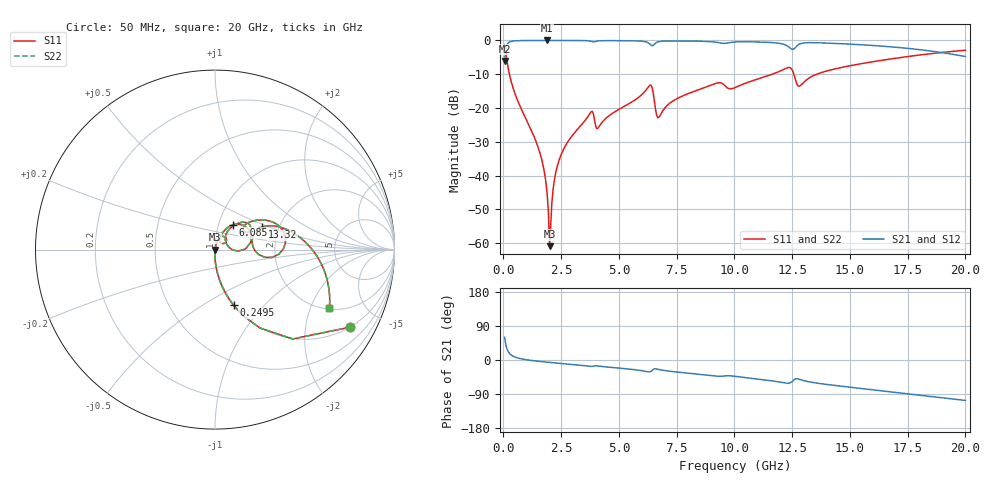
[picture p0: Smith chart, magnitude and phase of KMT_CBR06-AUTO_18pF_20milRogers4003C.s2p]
! Data measured by Modelithics Inc. support@modelithics.com 813-866-6335
! KEMET CBR06-AUTO 18pF, Pad Width= 0.851mm, Pad Length= 0.64mm, Pad Gap= 0.62mm, 20mil Rogers 4003C substrate Data, January 2022
# hz S ma R 50
! 2 Port Network Data from SP1.SP block
! freq  magS11  angS11  magS21  angS21  magS12  angS12  magS22  angS22
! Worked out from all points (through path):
!   401 points, 50 MHz to 20 GHz, reference 50 ohm
!   highest |S21| = -0.01 dB at 1.895 GHz (marker M1); lowest = -6.1 dB at 50 MHz (marker M2)
!   group delay of S21, straight-line fit = 15.3 ps
!   lowest |S11| = -60.8 dB at 1.995 GHz (marker M3), VSWR 1.00, Z = 50.1 - j0.0639 ohm
!   |S11| at or under -10 dB: 259.7 MHz to 11.63 GHz (11.37 GHz wide, 191 % of centre); 12.57 GHz to 13.56 GHz (987.4 MHz wide, 7.56 % of centre)
!   |S22| runs from -60.8 to -1.2 dB; largest |S21 - S12| = 0
!   S11 on the Smith chart (normalised r, x): 50 MHz: 0.99, -3.49; 249.5 MHz: 0.99, -0.69; 6.085 GHz: 1.17, +0.33; 13.32 GHz: 1.63, +0.44; 20 GHz: 2.04, -2.74
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5e7  0.8688 -29.8  0.4948 60.2  0.4948 60.2  0.8688 -29.8
2.495e8  0.3275 -71.6  0.9444 18.3  0.9444 18.3  0.3275 -71.6
1.596125e9  0.02067 -92.2  0.9991 -3.9  0.9991 -3.9  0.02067 -92.2
1.795625e9  0.01007 -91.3  0.9992 -5.2  0.9992 -5.2  0.01007 -91.3
1.895375e9  0.005236 -88.2  0.9992 -5.8  0.9992 -5.8  0.005236 -88.2
1.995125e9  0.0009071 -44.7  0.9992 -6.4  0.9992 -6.4  0.0009071 -44.7
2.2445e9  0.01027 77.9  0.9991 -7.8  0.9991 -7.8  0.01027 77.9
2.444e9  0.01835 78.6  0.9989 -8.9  0.9989 -8.9  0.01835 78.6
3.391625e9  0.05732 73.4  0.9958 -14.1  0.9958 -14.1  0.05732 73.4
3.790625e9  0.08773 57.2  0.9724 -17.0  0.9724 -17.0  0.08773 57.2
4.13975e9  0.05313 60.5  0.9863 -16.2  0.9863 -16.2  0.05313 60.5
6.084875e9  0.1704 54.1  0.9653 -29.1  0.9653 -29.1  0.1704 54.1
6.384125e9  0.218 23.0  0.8543 -30.4  0.8543 -30.4  0.218 23.0
6.73325e9  0.07323 34.3  0.9604 -25.0  0.9604 -25.0  0.07323 34.3
9.0275e9  0.2216 43.5  0.9552 -41.3  0.9552 -41.3  0.2216 43.5
1.0025e10  0.2006 37.8  0.9482 -43.1  0.9482 -43.1  0.2006 37.8
1.231925e10  0.3964 13.3  0.8176 -61.2  0.8176 -61.2  0.3964 13.3
1.2818e10  0.2109 11.2  0.8836 -51.0  0.8836 -51.0  0.2109 11.2
1.331675e10  0.2893 25.5  0.9268 -58.5  0.9268 -58.5  0.2893 25.5
1.336662e10  0.2954 25.4  0.9265 -59.0  0.9265 -59.0  0.2954 25.4
1.670825e10  0.5289 1.7  0.8079 -83.8  0.8079 -83.8  0.5289 1.7
2e10  0.7161 -27.1  0.5777 -106.6  0.5777 -106.6  0.7161 -27.1
